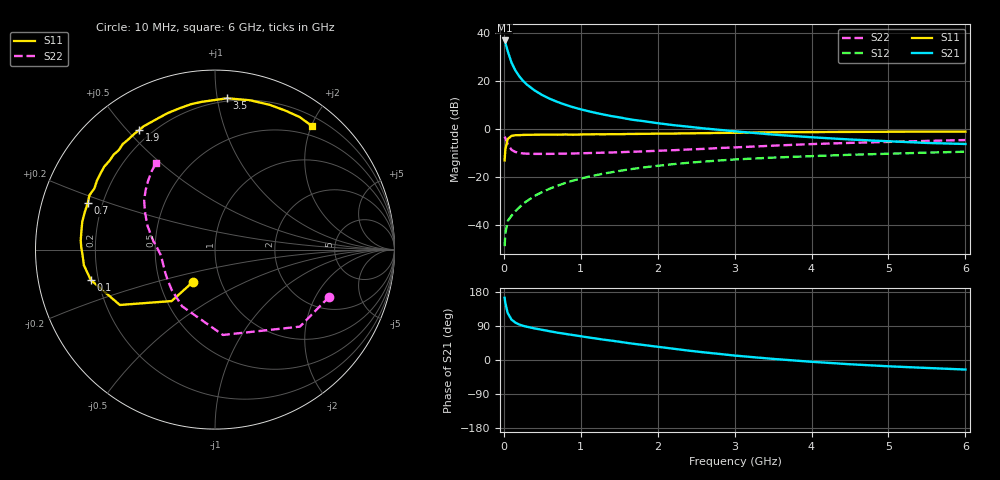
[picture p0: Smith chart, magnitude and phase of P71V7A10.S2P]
! SIEMENS Small Signal Semiconductors
! BFP196
! Si NPN RF Bipolar Junction Transistor in SOT143
! VCE = 1.75 V  IC = 100 mA
! Common Emitter S-Parameters:  May  1996
# GHz  S  MA  R  50
!  f  S11  S21  S12  S22
! GHz  MAG  ANG  MAG  ANG  MAG  ANG  MAG  ANG
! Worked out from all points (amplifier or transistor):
!   36 points, 10 MHz to 6 GHz, reference 50 ohm
!   highest |S21| = 36.8 dB at 10 MHz (marker M1)
!   |S21| within 3 dB of that: start of sweep to 37.66 MHz
!   unconditionally stable (mu >= 1): 233.9 MHz to end of sweep
!   at 250 MHz: K = 1.01, MAG = 24.9 dB, |S12| = -31.3 dB
!   at 1.4 GHz: K = 1.12, MAG = 9.6 dB, |S12| = -18.1 dB
!   at 6 GHz: K = 1.02, MAG = 0.7 dB, |S12| = -9.5 dB
!   S11 on the Smith chart (normalised r, x): 10 MHz: 0.73, -0.28; 100 MHz: 0.17, -0.12; 700 MHz: 0.14, +0.17; 1.9 GHz: 0.15, +0.54; 3.5 GHz: 0.18, +1.07; 6 GHz: 0.34, +2.00
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0.01  0.2202 -124.5  69.13 164.2  0.0036 70.7  0.6889 -22.3
0.02  0.3748 -130.1  62.03 149.7  0.0066 62.6  0.6388 -42.2
0.05  0.6134 -149.8  41.47 124.0  0.012 52.0  0.4776 -84.7
0.1  0.7125 -166.3  23.85 106.5  0.0156 51.4  0.3652 -120.1
0.15  0.7357 -173.2  16.41 98.7  0.0193 55.7  0.3294 -137.0
0.2  0.7386 -177.7  12.46 93.7  0.023 59.8  0.314 -146.9
0.25  0.7455 178.8  9.951 90.3  0.0273 61.8  0.3068 -153.7
0.3  0.7499 176.1  8.335 87.7  0.0313 64.2  0.3035 -157.7
0.4  0.7523 171.2  6.291 83.3  0.04 66.4  0.3003 -163.7
0.5  0.7557 168.0  5.037 79.6  0.0482 67.3  0.3001 -167.6
0.6  0.7549 163.8  4.203 75.7  0.057 67.1  0.3008 -170.1
0.7  0.7547 159.9  3.614 72.0  0.0655 66.7  0.3027 -172.2
0.9  0.7535 153.1  2.819 65.8  0.0836 64.7  0.306 -175.6
1.1  0.7659 146.5  2.325 59.5  0.1004 62.5  0.3127 -178.0
1.4  0.7738 136.8  1.838 51.1  0.1246 58.0  0.3214 178.6
1.9  0.7885 122.5  1.381 37.4  0.1628 50.1  0.3438 173.0
2.2  0.7961 114.5  1.194 29.9  0.1836 45.3  0.3584 169.1
2.8  0.8213 99.3  0.952 16.1  0.2191 35.9  0.3979 160.8
3.5  0.8459 85.4  0.758 2.9  0.2516 25.5  0.4457 151.3
4.5  0.8623 69.3  0.599 -11.2  0.2876 13.2  0.5091 139.4
5.5  0.8763 57.4  0.508 -21.0  0.3192 2.4  0.5597 129.3
6  0.8752 52.0  0.483 -25.2  0.3335 -3.5  0.5837 124.3
